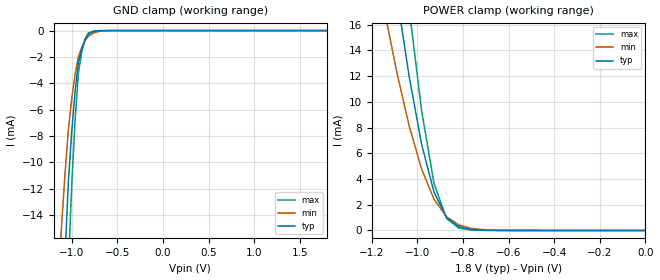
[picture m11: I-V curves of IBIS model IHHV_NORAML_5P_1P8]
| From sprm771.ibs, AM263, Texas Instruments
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|   Model Cell IHHV_NORAML_5P_1P8
|IHHV_NORAML_5P_1P8
[Model]   IHHV_NORAML_5P_1P8
Model_type   Input
Polarity   Non-Inverting
Vinl =  0.45
Vinh =  1.35
C_comp   0.8445658p   0.7268375p   1.0147853p
|[Input load] normal
|[supplytol] 5
|[temp] ind
[Model Spec]
Vinl   0.45   0.45   0.45
Vinh   1.35   1.35   1.35
[Temperature Range]   25   125   -40
[Voltage Range]   1.8   1.71   1.89
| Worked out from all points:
|   GND clamp passes 1 mA (typ) near -0.87 V on its own axis
|   POWER clamp passes 1 mA (typ) near -0.87 V on its own axis
| Nom Voltages:
|   VDD=1.1, VDDS=1.8, VDDS18=1.8, BUS_VSSS=0, ESD_BIASFET=0, VSS=0
| Min Voltages:
|   VDD=1.045, VDDS=1.71, VDDS18=1.71, BUS_VSSS=0, ESD_BIASFET=0, VSS=0
| Max Voltages:
|   VDD=1.16, VDDS=1.89, VDDS18=1.89, BUS_VSSS=0, ESD_BIASFET=0, VSS=0
[POWER_clamp]
|   voltage   I(typ)   I(min)   I(max)
-1.8V     125.2mA    90.57mA    173.6mA
-1.127V   23mA       15.53mA    33.25mA
-1.073V   16.2mA     10.93mA    23.45mA
-1.055V   14.09mA    9.536mA    20.36mA
-1.036V   11.97mA    8.138mA    17.26mA
-1.018V   10.21mA    7.016mA    14.61mA
-981.8mV  6.693mA    4.772mA    9.305mA
-927.3mV  2.976mA    2.421mA    3.639mA
-872.7mV  1.022mA    1.067mA    939uA
-818.2mV  292.9uA    424.1uA    183.7uA
-654.5mV  5.109uA    21.1uA     1.004uA
0V        63.92pA    193.7pA    203.8pA
[GND_clamp]
|   voltage   I(typ)   I(min)   I(max)
-1.8V     -188.2mA   -124.9mA   -283.5mA
-1.145V   -29.69mA   -18.67mA   -46.57mA
-1.109V   -22.95mA   -14.5mA    -35.97mA
-1.073V   -16.85mA   -10.76mA   -26.36mA
-1.036V   -11.41mA   -7.446mA   -17.74mA
-1V       -7.622mA   -5.159mA   -11.67mA
-963.6mV  -4.626mA   -3.338mA   -6.817mA
-927.3mV  -2.419mA   -1.986mA   -3.194mA
-890.9mV  -1.398mA   -1.289mA   -1.668mA
-818.2mV  -282uA     -434uA     -178.9uA
-600mV    -574.5nA   -6.687uA   -67.09nA
1.8V      0A         0A         0A
